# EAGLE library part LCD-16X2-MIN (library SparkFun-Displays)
RGB 16x2 parallel input LCD, 4bit only Basic 16 character by 2 line display. Typically utilizes the extremely common HD44780 parallel interface chipset SparkFun Products: Basic 16x2 RGB
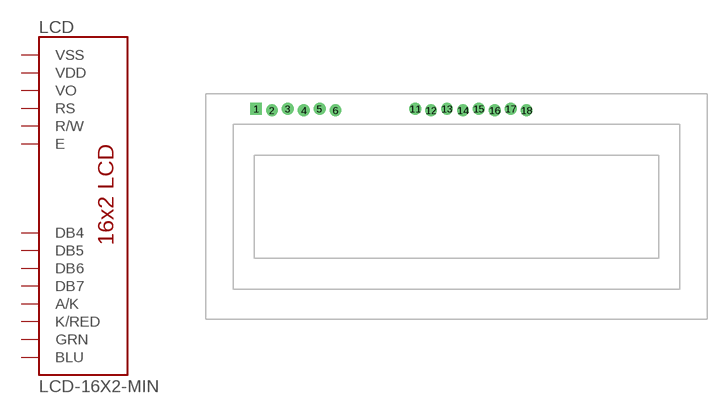
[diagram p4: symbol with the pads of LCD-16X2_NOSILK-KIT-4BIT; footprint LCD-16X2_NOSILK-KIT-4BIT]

Designator prefix LCD

## LCD-16X2-MINMIN4-RGB (SF_ID: LCD-10862)  [LCD-16X2_NOSILK-KIT-4BIT]
1  VSS  pwr
2  VDD  pwr
3  VO
4  RS  in
5  R/W  in
6  E  in
11  DB4
12  DB5
13  DB6
14  DB7
15  A/K  pwr
16  K/RED  pwr
17  GRN  pwr
18  BLU  pwr

## Footprint LCD-16X2_NOSILK-KIT-4BIT (pad centres in mm)
LCD-16x2, 4 bit for Kits For Standard hitatchi type LCDs with backlight. Has a gapped 16-pin connection and outline on docu, but no silk or mounting holes. Warning: This is the kit version of the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
drill 1.016 pad 1.88 square: 1 -32,15.627
drill 1.016 pad 1.88: 2 -29.46,15.373; 3 -26.92,15.627; 4 -24.38,15.373; 5 -21.84,15.627; 6 -19.3,15.373; 11 -6.6,15.627; 12 -4.06,15.373; 13 -1.52,15.627; 14 1.02,15.373; 15 3.56,15.627; 16 6.1,15.373; 17 8.64,15.627; 18 11.18,15.373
